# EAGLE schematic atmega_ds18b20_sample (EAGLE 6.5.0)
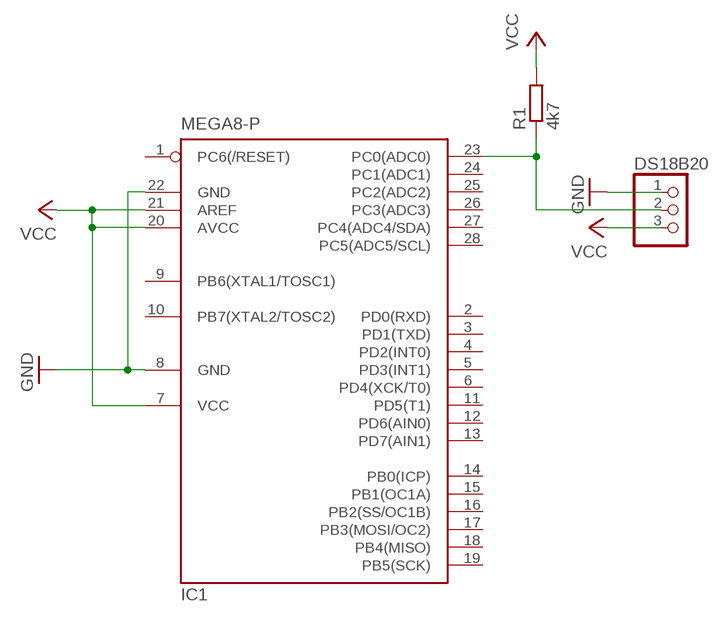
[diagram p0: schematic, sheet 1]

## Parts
DS18B20  PINHD-1X3  [1X03]
IC1  MEGA8-P  [DIL28-3]
R1  4k7  R-EU_0207/7  [0207/7]

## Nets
GND: DS18B20.1 IC1.8(GND) IC1.22(GND)
N$1: DS18B20.2 IC1.23(PC0(ADC0)) R1.1
VCC: DS18B20.3 IC1.7(VCC) IC1.20(AVCC) IC1.21(AREF) R1.2
Unconnected: IC1.1(PC6(/RESET)) IC1.2(PD0(RXD)) IC1.3(PD1(TXD)) IC1.4(PD2(INT0)) IC1.5(PD3(INT1)) IC1.6(PD4(XCK/T0)) IC1.9(PB6(XTAL1/TOSC1)) IC1.10(PB7(XTAL2/TOSC2)) IC1.11(PD5(T1)) IC1.12(PD6(AIN0)) IC1.13(PD7(AIN1)) IC1.14(PB0(ICP)) IC1.15(PB1(OC1A)) IC1.16(PB2(SS/OC1B)) IC1.17(PB3(MOSI/OC2)) IC1.18(PB4(MISO)) IC1.19(PB5(SCK)) IC1.24(PC1(ADC1)) IC1.25(PC2(ADC2)) IC1.26(PC3(ADC3)) IC1.27(PC4(ADC4/SDA)) IC1.28(PC5(ADC5/SCL))

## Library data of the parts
DS18B20 = pinhead:PINHD-1X3: PIN HEADER
IC1 = atmel:MEGA8-P: MICROCONTROLLER 8 Kbytes FLASH, 1 kbytes SRAM, 512 bytes EEPROM, USART, 4-channel 10 bit ADC, 2-channel 8 bit ADC Pin compatible with Atmega48, ATMega88, ATMega168 Source: avr.lbr
R1 = rcl:R-EU_: RESISTOR, European symbol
